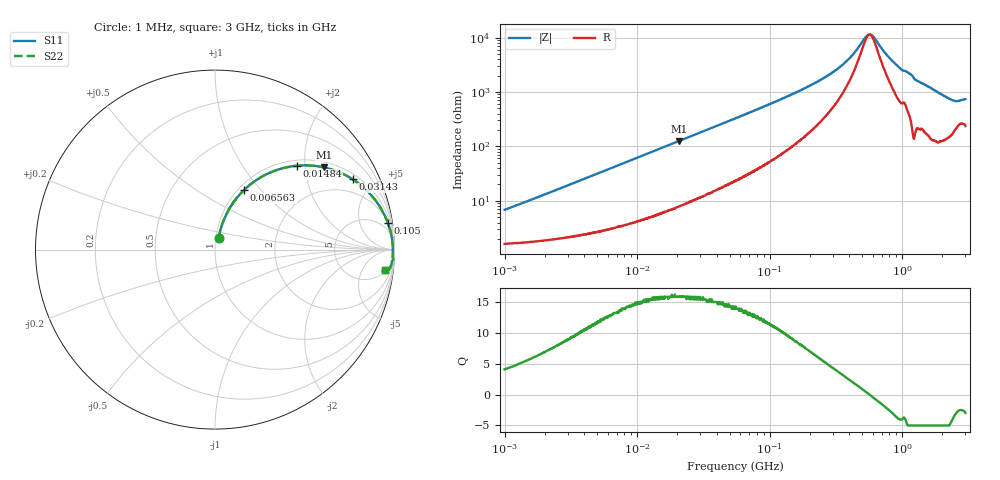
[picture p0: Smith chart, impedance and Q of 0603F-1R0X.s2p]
!s-Parameter Generated by FASTRON Sdn. Bhd.
!FASTRON P/N : 0603F-1R0X
!Keysight Technologies: E4991B_MY54100416_A.01.15
!Date: Wed Jun 19 15:37:14 2024
!Version  :Rev00  Wed Jun 19 15:37:14 2024
!Data & Calibration Information:
!Freq  S11  S21  S12  S22
!PortZ  Port1:50+j0  Port2:50+j0
!When reading reference impedance value at option line is always used.
! Remarks : This data is being provided solely for informational purposes.
# Hz S dB R 50
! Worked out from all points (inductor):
!   1601 points, 1 MHz to 3 GHz, reference 50 ohm
!   read as one part in series: L = 1.05 uH near 1.041 MHz
!   highest Q = 15.9 at 20.75 MHz (marker M1), where L = 965 nH
!   self-resonance near 568 MHz
!   S11 on the Smith chart (normalised r, x): 1 MHz: 1.03, +0.13; 6.563 MHz: 1.06, +0.82; 14.84 MHz: 1.12, +1.82; 31.43 MHz: 1.24, +3.76; 105 MHz: 2, +13; 3 GHz: 6, -14
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1000000  -23.40 72.6  -0.16 -3.8  -0.16 -3.8  -23.40 72.6
3804036  -12.70 71.2  -0.44 -13.3  -0.44 -13.3  -12.70 71.2
6563319  -8.62 63.9  -0.91 -21.7  -0.91 -21.7  -8.62 63.9
1.447069e7  -3.82 46.4  -2.79 -40.0  -2.79 -40.0  -3.82 46.4
1.483731e7  -3.71 45.7  -2.88 -40.6  -2.88 -40.6  -3.71 45.7
2.074721e7  -2.38 37.0  -4.39 -49.4  -4.39 -49.4  -2.38 37.0
3.142935e7  -1.30 27.1  -6.82 -59.3  -6.82 -59.3  -1.30 27.1
5.504702e7  -0.56 16.6  -10.90 -69.3  -10.90 -69.3  -0.56 16.6
1.049728e8  -0.23 8.9  -16.20 -76.0  -16.20 -76.0  -0.23 8.9
2.083556e8  -0.12 4.1  -22.80 -77.5  -22.80 -77.5  -0.12 4.1
3.541315e8  -0.09 1.7  -30.00 -71.1  -30.00 -71.1  -0.09 1.7
4.177151e8  -0.08 1.1  -33.40 -63.6  -33.40 -63.6  -0.08 1.1
5.232078e8  -0.08 0.3  -39.80 -29.9  -39.80 -29.9  -0.08 0.3
5.583748e8  -0.08 0.1  -41.10 -7.1  -41.10 -7.1  -0.08 0.1
6.079533e8  -0.08 -0.2  -40.30 26.0  -40.30 26.0  -0.08 -0.2
7.925923e8  -0.08 -1.2  -32.90 66.7  -32.90 66.7  -0.08 -1.2
9.682285e8  -0.08 -2.0  -28.70 74.1  -28.70 74.1  -0.08 -2.0
1.147801e9  -0.07 -2.6  -26.70 78.5  -26.70 78.5  -0.07 -2.6
1.281378e9  -0.08 -3.5  -24.30 79.2  -24.30 79.2  -0.08 -3.5
1.980367e9  -0.18 -6.2  -19.30 75.9  -19.30 75.9  -0.18 -6.2
2.468121e9  -0.42 -7.6  -17.20 66.4  -17.20 66.4  -0.42 -7.6
3e9  -0.43 -7.0  -17.80 64.3  -17.80 64.3  -0.43 -7.0
